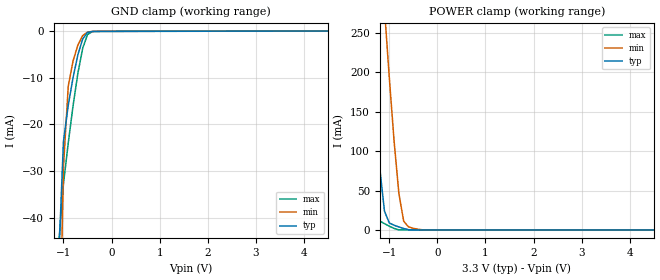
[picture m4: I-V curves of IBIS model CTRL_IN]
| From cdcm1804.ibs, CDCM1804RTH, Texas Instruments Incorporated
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| Device Control Input
[Model]   CTRL_IN
Model_type  Input
Polarity   Non-Inverting
Vinl = 0.8V
Vinh = 2.0V
| variable   typ   min   max
C_comp   0.57p   NA   NA
[Temperature Range]   27   125   -20
[Voltage range]   3.3   3.0   3.6
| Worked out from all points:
|   GND clamp passes 1 mA (typ) near -0.55 V on its own axis
|   POWER clamp passes 1 mA (typ) near -0.64 V on its own axis
|Process range|   nominal   weak   strong
[POWER Clamp]
|   27C:3.3V:nominal   125C:3.0V:weak   -20C:3.6V:strong
|  Voltage   I(typ)   I(min)   I(max)
-3.6V     2.38A      2.7A       2.08A
-1.8V     621mA      939mA      320mA
-1.7V     526mA      842mA      228mA
-1.5V     338mA      651mA      63.3mA
-1.4V     247mA      557mA      21.9mA
-1.2V     80.2mA     371mA      11.5mA
-1.1V     24mA       281mA      8.03mA
-900mV    6mA        113mA      1.98mA
-800mV    3.83mA     46.4mA     107uA
-700mV    1.92mA     11.1mA     18.2uA
-500mV    47.1uA     2.12mA     3.93uA
6.6V      0A         0A         0A
[GND Clamp]
|   27C:3.3V:nominal   125C:3.0V:weak   -20C:3.6V:strong
|  Voltage   I(typ)   I(min)   I(max)
-3.7V     -2.52A     -2.55A     -2.5A
-1.1V     -49.4mA    -79.5mA    -45.7mA
-1V       -23.7mA    -29.2mA    -32.8mA
-900mV    -15.9mA    -11.8mA    -24mA
-800mV    -9.97mA    -6.41mA    -16mA
-700mV    -5.09mA    -3.01mA    -9.06mA
-600mV    -1.7mA     -962uA     -3.7mA
-500mV    -307uA     -216uA     -748uA
-400mV    -81.4uA    -73.6uA    -118uA
-300mV    -62.2uA    -54uA      -77.5uA
6.6V      0A         0A         0A
